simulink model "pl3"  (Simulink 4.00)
settings: Solver=ode45  StartTime=0.0  StopTime=8  RelTol=1e-3
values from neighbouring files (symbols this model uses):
  m = p    (= 10)    [scr1.m]    (also in scrmod1.m; scr.m; Smpc.m = mp(1:max(size(mp))-1); demo1dat.m = 4)
  model = tfd2step(tfinal,Ts,1,g)    [scr1.m]    (also in scrmod1.m = [y(2:ly); 1; 1; .1]; scr.m = [y(2:ly); 1; 1; .1]; Smpc.m = modelpd(:,1:nu); essai2dat.m = tfd2step(1.6,delt,1,g))
  p = 10    [scr1.m]    (also in scrmod1.m; scr.m; Smpc.m = mp(max(size(mp))); demo1dat.m)
  Ts = .1    (= 0.1)    [scr1.m]    (also in scrmod1.m; Smpc.m = [tsamp 0]; mynlcmpc.m = [tsamp 0]; mynlcmpc2.m = [tsamp 0])
  ulim = [-4 4 .5]    [scr1.m]    (also in scrmod1.m = []; scr.m; Smpc.m = [-inf*ones(1,nu) inf*ones(1,nu) 1e6*ones(1,nu)]; essai2dat.m = [-5 40 3])
  uwt = 1    [scr1.m]    (also in scrmod1.m; scr.m; Smpc.m = yuwt(:,ny+1:ny+nu); demo1dat.m = [0 0])
  ylim = [-inf inf]    [scr1.m]    (also in scrmod1.m = []; scr.m; Smpc.m = [ylim; ylim(N,:)]; essai2dat.m = [-40 40])
  ywt = 5    [scr1.m]    (also in scrmod1.m; scr.m; Smpc.m = yuwt(:,1:ny); demo1dat.m = [1 1])

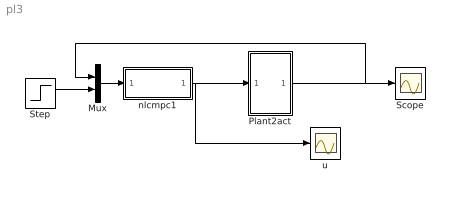
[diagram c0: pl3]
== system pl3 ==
  Mux : Mux  Inputs=2
  Plant2act : Subsystem
  Scope : Scope
  Step : Step  Time=1  Before=0  After=1  SampleTime=0
  nlcmpc1 : Subsystem  AncestorBlock=nlmpclib/nlcmpc  mask(Smpc){modelpd=[model []], yuwt=[ywt uwt], mp=[m p], yulim=[ylim ulim], tfilter=[], ud0=[0 []]}
      mask help: Masked MATLAB function block calls nlcmpc, links CMPC and SIMULINK.
  u : Scope
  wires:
  Plant2act/1(y) -> Scope/1, Mux/1
  nlcmpc1/1(Out1) -> u/1, Plant2act/1(u)
  Mux/1 -> nlcmpc1/1(In1)
  Step/1 -> Mux/2

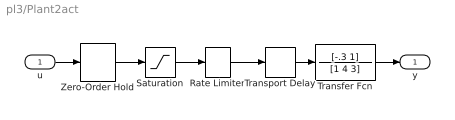
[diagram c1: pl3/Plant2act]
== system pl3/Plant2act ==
  u : Inport  Port=1  LatchInput=off
  Rate Limiter : RateLimiter  RisingSlewLimit=1/Ts  FallingSlewLimit=-1/Ts
  Saturation : Saturate  UpperLimit=2  LowerLimit=-2  LinearizeAsGain=on
  Transfer Fcn : TransferFcn  Numerator=[-.3 1]  Denominator=[1 4 3]  AbsoluteTolerance=auto  Realization=auto
  Transport Delay : TransportDelay  DelayTime=.2  InitialInput=0  BufferSize=1024  PadeOrder=0
  Zero-Order Hold : ZeroOrderHold  SampleTime=0.1
  y : Outport  Port=1
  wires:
  Transport Delay/1 -> Transfer Fcn/1
  u/1 -> Zero-Order Hold/1
  Transfer Fcn/1 -> y/1
  Saturation/1 -> Rate Limiter/1
  Zero-Order Hold/1 -> Saturation/1
  Rate Limiter/1 -> Transport Delay/1

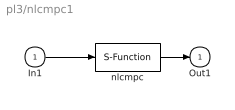
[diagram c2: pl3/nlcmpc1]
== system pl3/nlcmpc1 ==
  In1 : Inport  Port=1  LatchInput=off
  nlcmpc : S-Function  FunctionName=Smpc  Parameters=modelpd,mp,tfilter,yuwt,ud0,yulim  PortCounts=[]  SFunctionModules=''
  Out1 : Outport  Port=1  InitialOutput=0
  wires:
  In1/1 -> nlcmpc/1
  nlcmpc/1 -> Out1/1
